FUNCTION "GESTIONE_ES" : VOID
TITLE =
{ S7_language := '9(1) Inglese (Stati Uniti)  21.12.2021  10:54:11' }
VERSION : 0.1


VAR_TEMP
  RETVAL : INT ;
END_VAR
BEGIN
NETWORK
TITLE =**************************************

NETWORK
TITLE =Abilita Gestione Risparmio Energetico
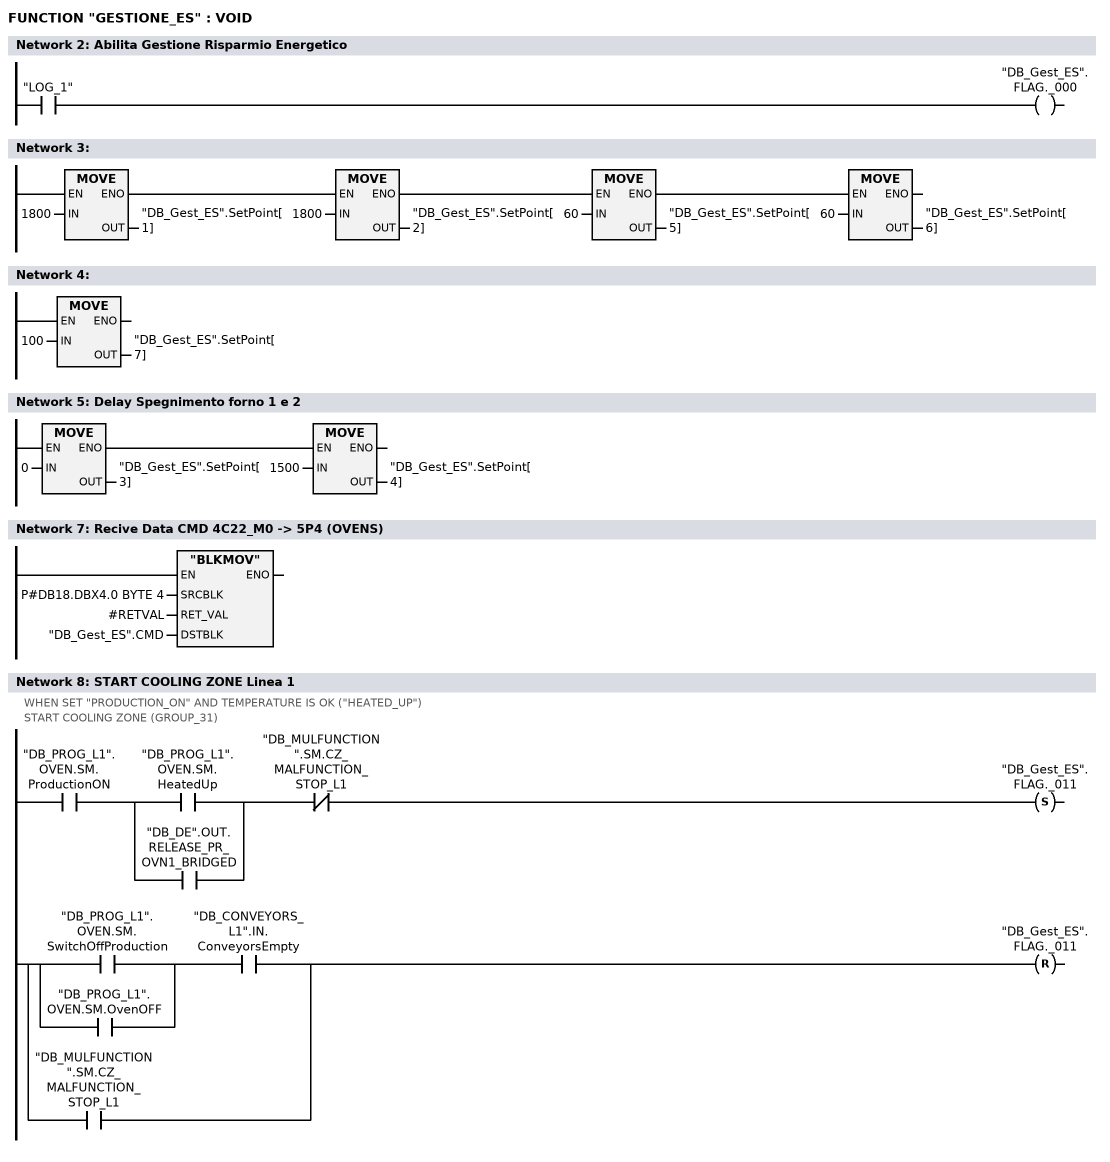
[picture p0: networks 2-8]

      U     "LOG_1";
      =     "DB_Gest_ES".FLAG._000;
NETWORK
TITLE =

      U(    ;
      U(    ;
      U(    ;
      L     1800;
      T     "DB_Gest_ES".SetPoint[1];
      SET   ;
      SAVE  ;
      CLR   ;
      U     BIE;
      )     ;
      SPBNB _001;
      L     1800;
      T     "DB_Gest_ES".SetPoint[2];
      SET   ;
      SAVE  ;
      CLR   ;
_001: U     BIE;
      )     ;
      SPBNB _002;
      L     60;
      T     "DB_Gest_ES".SetPoint[5];
      SET   ;
      SAVE  ;
      CLR   ;
_002: U     BIE;
      )     ;
      SPBNB _003;
      L     60;
      T     "DB_Gest_ES".SetPoint[6];
_003: NOP   0;
NETWORK
TITLE =

      L     100;
      T     "DB_Gest_ES".SetPoint[7];
      NOP   0;
NETWORK
TITLE =Delay Spegnimento forno 1 e 2

      U(    ;
      L     0;
      T     "DB_Gest_ES".SetPoint[3];
      SET   ;
      SAVE  ;
      CLR   ;
      U     BIE;
      )     ;
      SPBNB _004;
      L     1500;
      T     "DB_Gest_ES".SetPoint[4];
_004: NOP   0;
NETWORK
TITLE =**************************************

NETWORK
TITLE =Recive Data CMD 4C22_M0 -> 5P4 (OVENS)

      CALL "BLKMOV" (
           SRCBLK                   := P#DB18.DBX4.0 BYTE 4,
           RET_VAL                  := #RETVAL,
           DSTBLK                   := "DB_Gest_ES".CMD);
      NOP   0;
NETWORK
TITLE =START COOLING ZONE Linea 1
//WHEN SET "PRODUCTION_ON" AND TEMPERATURE IS OK ("HEATED_UP")
//START COOLING ZONE (GROUP_31)
      U     "DB_PROG_L1".OVEN.SM.ProductionON;
      U(    ;
      O     "DB_PROG_L1".OVEN.SM.HeatedUp;
      O     "DB_DE".OUT.RELEASE_PR_OVN1_BRIDGED;
      )     ;
      UN    "DB_MULFUNCTION".SM.CZ_MALFUNCTION_STOP_L1;
      S     "DB_Gest_ES".FLAG._011;
      U(    ;
      U(    ;
      O     "DB_PROG_L1".OVEN.SM.SwitchOffProduction;
      O     "DB_PROG_L1".OVEN.SM.OvenOFF;
      )     ;
      U     "DB_CONVEYORS_L1".IN.ConveyorsEmpty;
      O     "DB_MULFUNCTION".SM.CZ_MALFUNCTION_STOP_L1;
      )     ;
      R     "DB_Gest_ES".FLAG._011;
      NOP   0;
NETWORK
TITLE =Stop Raffreddamento Linea 1
//DB8.DBD38
      U     "DB_Gest_ES".FLAG._011;
      U     "DB_Gest_ES".FLAG._000;
      =     L      2.0;
      U     L      2.0;
      U(    ;
      U     "DB_Gest_ES".CMD.StopVentilazione_Zona1;
      UN    "DB_Gest_ES".FLAG._013;
      O     ;
      U     "DB_Gest_ES".Tmr.EN_Delay_01;
      UN    "DB_Gest_ES".Tmr.DN_Delay_01;
      )     ;
      S     "DB_Gest_ES".FLAG._001;
      U     L      2.0;
      UN    "DB_Gest_ES".CMD.StopVentilazione_Zona1;
      UN    "DB_Gest_ES".FLAG._013;
      S     "DB_Gest_ES".FLAG._013;
      U(    ;
      U     L      2.0;
      U     "DB_Gest_ES".CMD.VentilazioneRid_Zona1;
      =     "DB_Gest_ES".Tmr.EN_Delay_05;
      U     "DB_Gest_ES".Tmr.EN_Delay_05;
      )     ;
      U     "DB_Gest_ES".Tmr.DN_Delay_05;
      =     "DB_Gest_ES".FLAG._021;
NETWORK
TITLE =AUX Start Raff. Linea 1
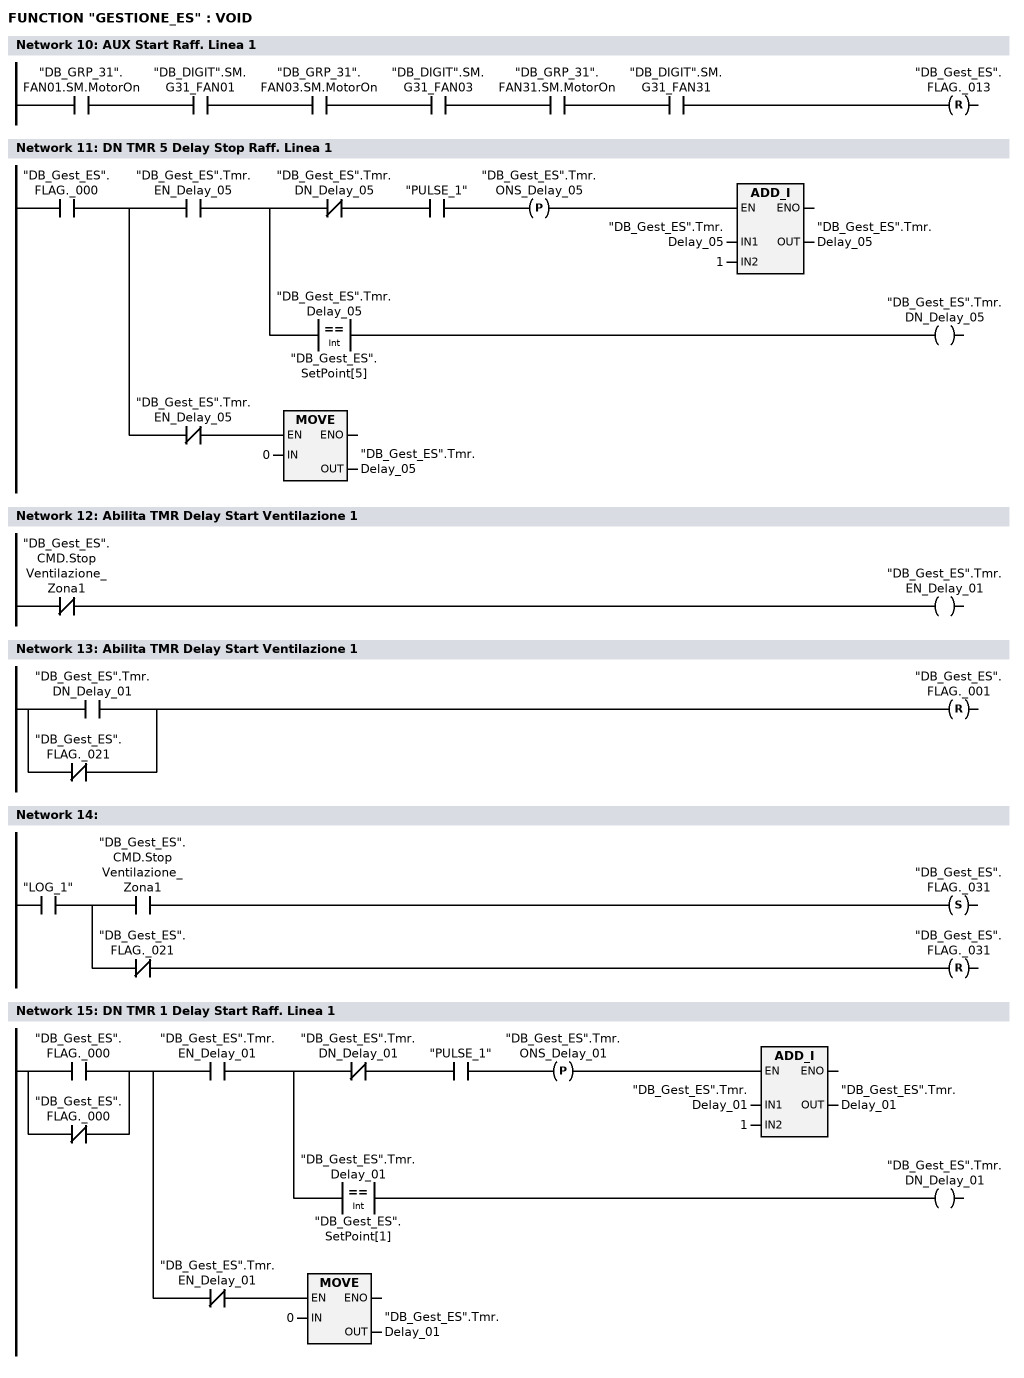
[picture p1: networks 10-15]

      U     "DB_GRP_31".FAN01.SM.MotorOn;
      U     "DB_DIGIT".SM.G31_FAN01;
      U     "DB_GRP_31".FAN03.SM.MotorOn;
      U     "DB_DIGIT".SM.G31_FAN03;
      U     "DB_GRP_31".FAN31.SM.MotorOn;
      U     "DB_DIGIT".SM.G31_FAN31;
      R     "DB_Gest_ES".FLAG._013;
NETWORK
TITLE =DN TMR 5 Delay Stop Raff. Linea 1

      U     "DB_Gest_ES".FLAG._000;
      =     L      2.0;
      U     L      2.0;
      U     "DB_Gest_ES".Tmr.EN_Delay_05;
      =     L      2.1;
      U     L      2.1;
      UN    "DB_Gest_ES".Tmr.DN_Delay_05;
      U     "PULSE_1";
      FP    "DB_Gest_ES".Tmr.ONS_Delay_05;
      SPBNB _005;
      L     "DB_Gest_ES".Tmr.Delay_05;
      L     1;
      +I    ;
      T     "DB_Gest_ES".Tmr.Delay_05;
_005: NOP   0;
      U     L      2.1;
      U(    ;
      L     "DB_Gest_ES".Tmr.Delay_05;
      L     "DB_Gest_ES".SetPoint[5];
      ==I   ;
      )     ;
      =     "DB_Gest_ES".Tmr.DN_Delay_05;
      U     L      2.0;
      UN    "DB_Gest_ES".Tmr.EN_Delay_05;
      SPBNB _006;
      L     0;
      T     "DB_Gest_ES".Tmr.Delay_05;
_006: NOP   0;
NETWORK
TITLE =Abilita TMR Delay Start Ventilazione 1

      UN    "DB_Gest_ES".CMD.StopVentilazione_Zona1;
      =     "DB_Gest_ES".Tmr.EN_Delay_01;
NETWORK
TITLE =Abilita TMR Delay Start Ventilazione 1

      O     "DB_Gest_ES".Tmr.DN_Delay_01;
      ON    "DB_Gest_ES".FLAG._021;
      R     "DB_Gest_ES".FLAG._001;
NETWORK
TITLE =

      U     "LOG_1";
      =     L      2.0;
      U     L      2.0;
      U     "DB_Gest_ES".CMD.StopVentilazione_Zona1;
      S     "DB_Gest_ES".FLAG._031;
      U     L      2.0;
      UN    "DB_Gest_ES".FLAG._021;
      R     "DB_Gest_ES".FLAG._031;
NETWORK
TITLE =DN TMR 1 Delay Start Raff. Linea 1

      O     "DB_Gest_ES".FLAG._000;
      ON    "DB_Gest_ES".FLAG._000;
      =     L      2.0;
      U     L      2.0;
      U     "DB_Gest_ES".Tmr.EN_Delay_01;
      =     L      2.1;
      U     L      2.1;
      UN    "DB_Gest_ES".Tmr.DN_Delay_01;
      U     "PULSE_1";
      FP    "DB_Gest_ES".Tmr.ONS_Delay_01;
      SPBNB _007;
      L     "DB_Gest_ES".Tmr.Delay_01;
      L     1;
      +I    ;
      T     "DB_Gest_ES".Tmr.Delay_01;
_007: NOP   0;
      U     L      2.1;
      U(    ;
      L     "DB_Gest_ES".Tmr.Delay_01;
      L     "DB_Gest_ES".SetPoint[1];
      ==I   ;
      )     ;
      =     "DB_Gest_ES".Tmr.DN_Delay_01;
      U     L      2.0;
      UN    "DB_Gest_ES".Tmr.EN_Delay_01;
      SPBNB _008;
      L     0;
      T     "DB_Gest_ES".Tmr.Delay_01;
_008: NOP   0;
NETWORK
TITLE =Stop Riscaldamento Linea 1

      U     "LOG_1";
      =     L      2.0;
      U(    ;
      U     L      2.0;
      U     "DB_Gest_ES".FLAG._000;
      U     "DB_CalendarioF1".CMD_OFF;
      U     "DB_CalendarioF1".Auto;
      UN    "DB_PROG_L1".OVEN.SM.SwitchOffProduction;
      U     "DB_Gest_ES".CMD.Stop_Riscarldo_Forno1;
      U     "DB_Gest_ES".CMD.AssenzaScoccheCabina;
      =     "DB_Gest_ES".Tmr.EN_Delay_03;
      U     "DB_Gest_ES".Tmr.EN_Delay_03;
      )     ;
      U     "DB_Gest_ES".Tmr.DN_Delay_03;
      S     "DB_Gest_ES".FLAG._003;
      R     "DB_CalendarioF1".CMD_OFF;
      U     L      2.0;
      U(    ;
      O     "DB_PROG_L1".OVEN.SM.SwitchOffProduction;
      O     "DB_PROG_L1".OVEN.SM.OvenOFF;
      O     "DB_PROG_L1".OVEN.CTRL.PreHeatingOn;
      O     "DB_PROG_L1".OVEN.CTRL.ProductionOn;
      )     ;
      R     "DB_Gest_ES".FLAG._003;
NETWORK
TITLE =DN TMR 3 Delay Stop Riscaldamento Linea 1
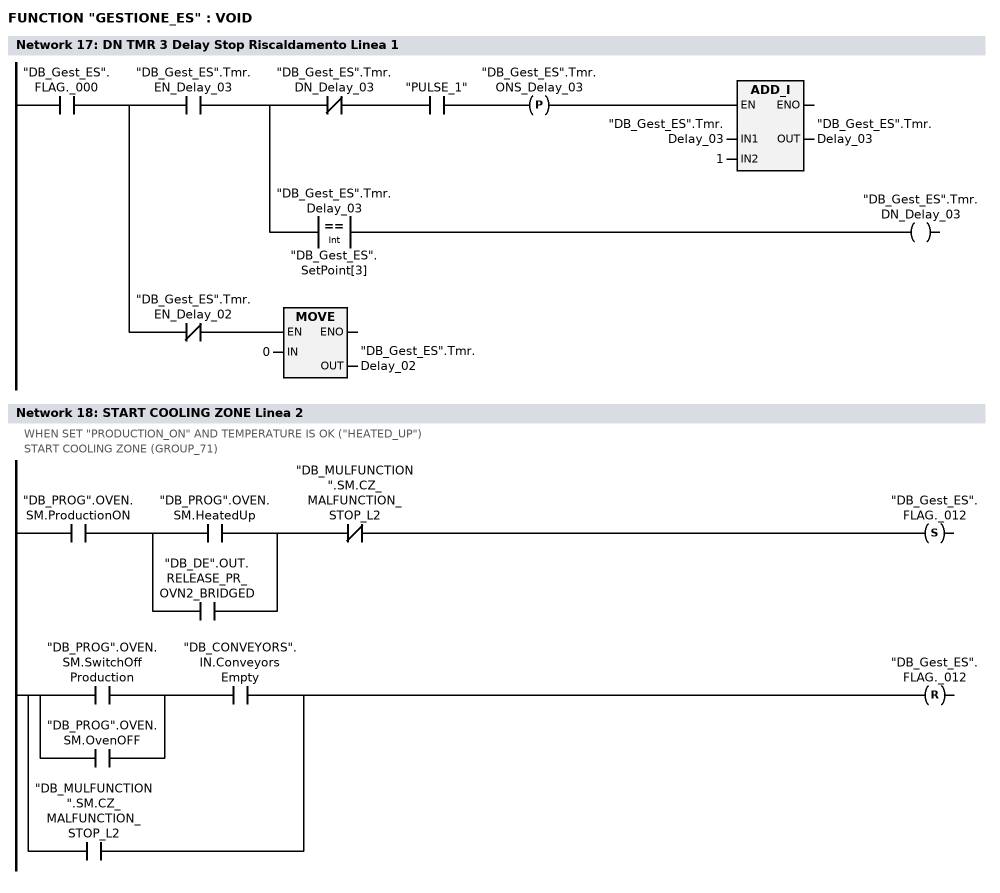
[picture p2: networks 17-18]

      U     "DB_Gest_ES".FLAG._000;
      =     L      2.0;
      U     L      2.0;
      U     "DB_Gest_ES".Tmr.EN_Delay_03;
      =     L      2.1;
      U     L      2.1;
      UN    "DB_Gest_ES".Tmr.DN_Delay_03;
      U     "PULSE_1";
      FP    "DB_Gest_ES".Tmr.ONS_Delay_03;
      SPBNB _009;
      L     "DB_Gest_ES".Tmr.Delay_03;
      L     1;
      +I    ;
      T     "DB_Gest_ES".Tmr.Delay_03;
_009: NOP   0;
      U     L      2.1;
      U(    ;
      L     "DB_Gest_ES".Tmr.Delay_03;
      L     "DB_Gest_ES".SetPoint[3];
      ==I   ;
      )     ;
      =     "DB_Gest_ES".Tmr.DN_Delay_03;
      U     L      2.0;
      UN    "DB_Gest_ES".Tmr.EN_Delay_02;
      SPBNB _00a;
      L     0;
      T     "DB_Gest_ES".Tmr.Delay_02;
_00a: NOP   0;
NETWORK
TITLE =START COOLING ZONE Linea 2
//WHEN SET "PRODUCTION_ON" AND TEMPERATURE IS OK ("HEATED_UP")
//START COOLING ZONE (GROUP_71)
      U     "DB_PROG".OVEN.SM.ProductionON;
      U(    ;
      O     "DB_PROG".OVEN.SM.HeatedUp;
      O     "DB_DE".OUT.RELEASE_PR_OVN2_BRIDGED;
      )     ;
      UN    "DB_MULFUNCTION".SM.CZ_MALFUNCTION_STOP_L2;
      S     "DB_Gest_ES".FLAG._012;
      U(    ;
      U(    ;
      O     "DB_PROG".OVEN.SM.SwitchOffProduction;
      O     "DB_PROG".OVEN.SM.OvenOFF;
      )     ;
      U     "DB_CONVEYORS".IN.ConveyorsEmpty;
      O     "DB_MULFUNCTION".SM.CZ_MALFUNCTION_STOP_L2;
      )     ;
      R     "DB_Gest_ES".FLAG._012;
      NOP   0;
NETWORK
TITLE =Stop Raffreddamento Linea 2
//DB8.DBD38
      U     "DB_Gest_ES".FLAG._012;
      U     "DB_Gest_ES".FLAG._000;
      =     L      2.0;
      U     L      2.0;
      U(    ;
      U     "DB_Gest_ES".CMD.StopVentilazione_Zona2;
      UN    "DB_Gest_ES".FLAG._014;
      O     ;
      U     "DB_Gest_ES".Tmr.EN_Delay_02;
      UN    "DB_Gest_ES".Tmr.DN_Delay_02;
      )     ;
      S     "DB_Gest_ES".FLAG._002;
      U     L      2.0;
      UN    "DB_Gest_ES".CMD.StopVentilazione_Zona2;
      UN    "DB_Gest_ES".FLAG._014;
      S     "DB_Gest_ES".FLAG._014;
      U(    ;
      U     L      2.0;
      U     "DB_Gest_ES".CMD.VentilazioneRid_Zona2;
      =     "DB_Gest_ES".Tmr.EN_Delay_06;
      U     "DB_Gest_ES".Tmr.EN_Delay_06;
      )     ;
      U     "DB_Gest_ES".Tmr.DN_Delay_06;
      =     "DB_Gest_ES".FLAG._022;
NETWORK
TITLE =AUX Start Raff. Linea 2
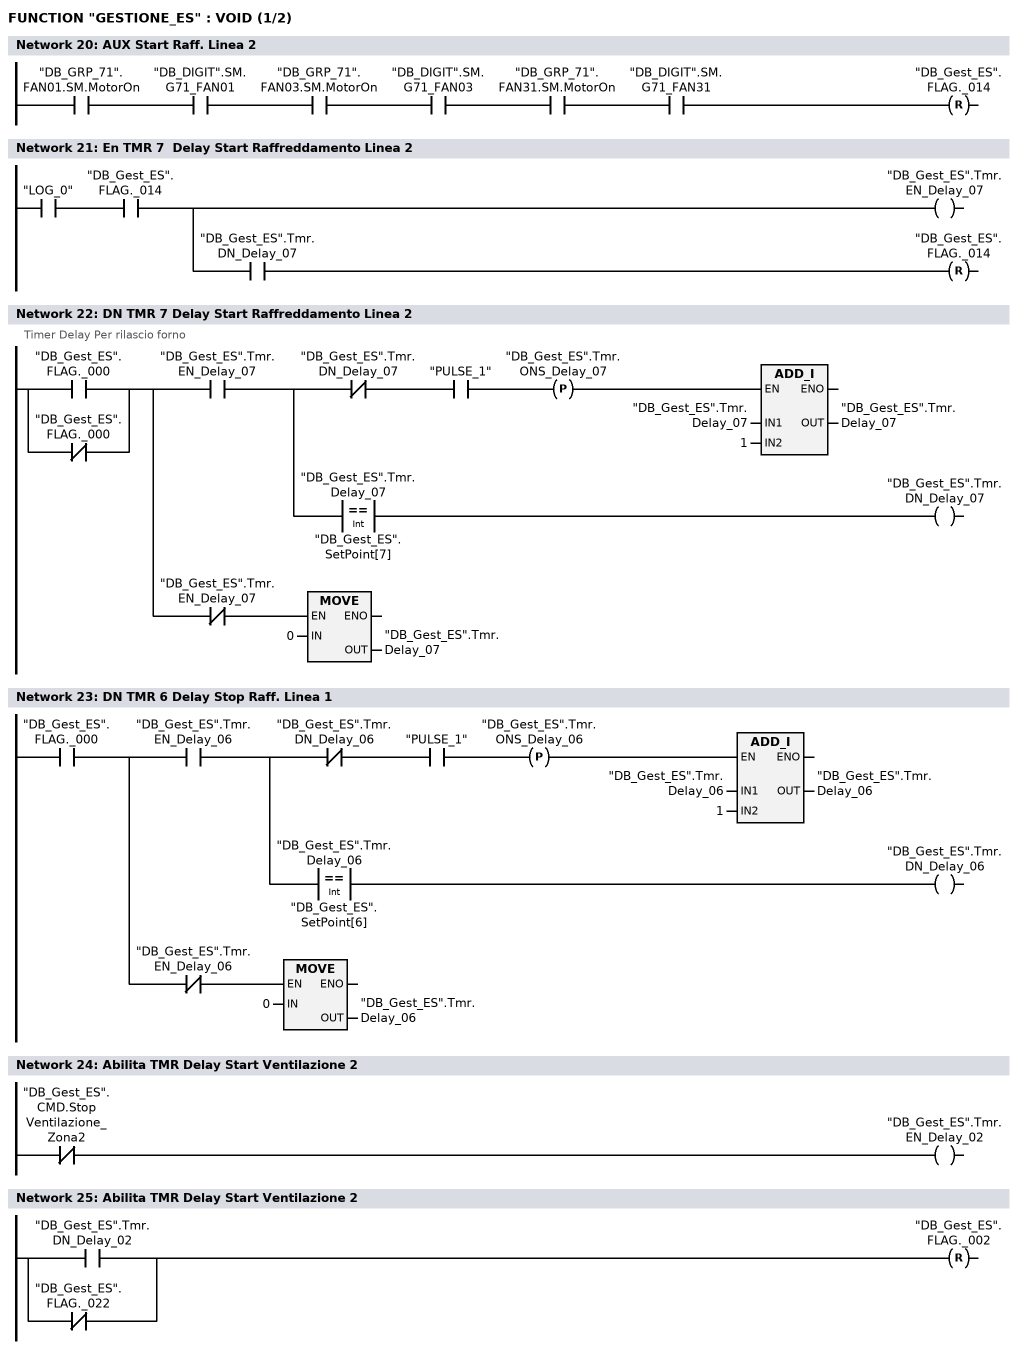
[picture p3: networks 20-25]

      U     "DB_GRP_71".FAN01.SM.MotorOn;
      U     "DB_DIGIT".SM.G71_FAN01;
      U     "DB_GRP_71".FAN03.SM.MotorOn;
      U     "DB_DIGIT".SM.G71_FAN03;
      U     "DB_GRP_71".FAN31.SM.MotorOn;
      U     "DB_DIGIT".SM.G71_FAN31;
      R     "DB_Gest_ES".FLAG._014;
NETWORK
TITLE =En TMR 7  Delay Start Raffreddamento Linea 2

      U     "LOG_0";
      U     "DB_Gest_ES".FLAG._014;
      =     L      2.0;
      U     L      2.0;
      BLD   102;
      =     "DB_Gest_ES".Tmr.EN_Delay_07;
      U     L      2.0;
      U     "DB_Gest_ES".Tmr.DN_Delay_07;
      R     "DB_Gest_ES".FLAG._014;
NETWORK
TITLE =DN TMR 7 Delay Start Raffreddamento Linea 2
//Timer Delay Per rilascio forno
      O     "DB_Gest_ES".FLAG._000;
      ON    "DB_Gest_ES".FLAG._000;
      =     L      2.0;
      U     L      2.0;
      U     "DB_Gest_ES".Tmr.EN_Delay_07;
      =     L      2.1;
      U     L      2.1;
      UN    "DB_Gest_ES".Tmr.DN_Delay_07;
      U     "PULSE_1";
      FP    "DB_Gest_ES".Tmr.ONS_Delay_07;
      SPBNB _00b;
      L     "DB_Gest_ES".Tmr.Delay_07;
      L     1;
      +I    ;
      T     "DB_Gest_ES".Tmr.Delay_07;
_00b: NOP   0;
      U     L      2.1;
      U(    ;
      L     "DB_Gest_ES".Tmr.Delay_07;
      L     "DB_Gest_ES".SetPoint[7];
      ==I   ;
      )     ;
      =     "DB_Gest_ES".Tmr.DN_Delay_07;
      U     L      2.0;
      UN    "DB_Gest_ES".Tmr.EN_Delay_07;
      SPBNB _00c;
      L     0;
      T     "DB_Gest_ES".Tmr.Delay_07;
_00c: NOP   0;
NETWORK
TITLE =DN TMR 6 Delay Stop Raff. Linea 1

      U     "DB_Gest_ES".FLAG._000;
      =     L      2.0;
      U     L      2.0;
      U     "DB_Gest_ES".Tmr.EN_Delay_06;
      =     L      2.1;
      U     L      2.1;
      UN    "DB_Gest_ES".Tmr.DN_Delay_06;
      U     "PULSE_1";
      FP    "DB_Gest_ES".Tmr.ONS_Delay_06;
      SPBNB _00d;
      L     "DB_Gest_ES".Tmr.Delay_06;
      L     1;
      +I    ;
      T     "DB_Gest_ES".Tmr.Delay_06;
_00d: NOP   0;
      U     L      2.1;
      U(    ;
      L     "DB_Gest_ES".Tmr.Delay_06;
      L     "DB_Gest_ES".SetPoint[6];
      ==I   ;
      )     ;
      =     "DB_Gest_ES".Tmr.DN_Delay_06;
      U     L      2.0;
      UN    "DB_Gest_ES".Tmr.EN_Delay_06;
      SPBNB _00e;
      L     0;
      T     "DB_Gest_ES".Tmr.Delay_06;
_00e: NOP   0;
NETWORK
TITLE =Abilita TMR Delay Start Ventilazione 2

      UN    "DB_Gest_ES".CMD.StopVentilazione_Zona2;
      =     "DB_Gest_ES".Tmr.EN_Delay_02;
NETWORK
TITLE =Abilita TMR Delay Start Ventilazione 2

      O     "DB_Gest_ES".Tmr.DN_Delay_02;
      ON    "DB_Gest_ES".FLAG._022;
      R     "DB_Gest_ES".FLAG._002;
NETWORK
TITLE =DN TMR 2 Delay Stop Riscaldamento Linea 2
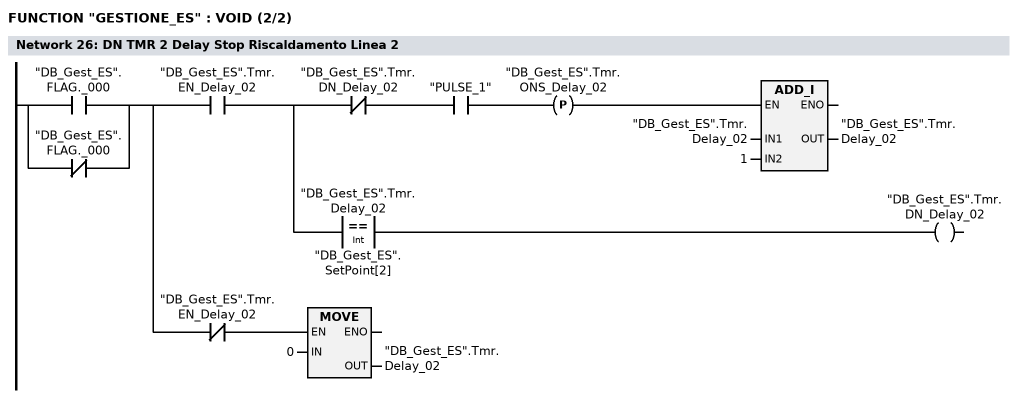
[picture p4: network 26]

      O     "DB_Gest_ES".FLAG._000;
      ON    "DB_Gest_ES".FLAG._000;
      =     L      2.0;
      U     L      2.0;
      U     "DB_Gest_ES".Tmr.EN_Delay_02;
      =     L      2.1;
      U     L      2.1;
      UN    "DB_Gest_ES".Tmr.DN_Delay_02;
      U     "PULSE_1";
      FP    "DB_Gest_ES".Tmr.ONS_Delay_02;
      SPBNB _00f;
      L     "DB_Gest_ES".Tmr.Delay_02;
      L     1;
      +I    ;
      T     "DB_Gest_ES".Tmr.Delay_02;
_00f: NOP   0;
      U     L      2.1;
      U(    ;
      L     "DB_Gest_ES".Tmr.Delay_02;
      L     "DB_Gest_ES".SetPoint[2];
      ==I   ;
      )     ;
      =     "DB_Gest_ES".Tmr.DN_Delay_02;
      U     L      2.0;
      UN    "DB_Gest_ES".Tmr.EN_Delay_02;
      SPBNB _010;
      L     0;
      T     "DB_Gest_ES".Tmr.Delay_02;
_010: NOP   0;
NETWORK
TITLE =Stop Riscaldamento Linea 2

      U     "LOG_1";
      =     L      2.0;
      U(    ;
      U     L      2.0;
      U     "DB_Gest_ES".FLAG._000;
      U     "DB_CalendarioF2".CMD_OFF;
      U     "DB_CalendarioF2".Auto;
      UN    "DB_PROG".OVEN.SM.SwitchOffProduction;
      U     "DB_Gest_ES".CMD.AssenzaScoccheCabina;
      =     "DB_Gest_ES".Tmr.EN_Delay_04;
      U     "DB_Gest_ES".Tmr.EN_Delay_04;
      )     ;
      U     "DB_Gest_ES".CMD.Stop_Riscarldo_Forno2;
      U     "DB_Gest_ES".Tmr.DN_Delay_04;
      S     "DB_Gest_ES".FLAG._004;
      R     "DB_CalendarioF2".CMD_OFF;
      U     L      2.0;
      U(    ;
      O     "DB_PROG".OVEN.SM.SwitchOffProduction;
      O     "DB_PROG".OVEN.SM.OvenOFF;
      O     "DB_PROG".OVEN.CTRL.PreHeatingOn;
      O     "DB_PROG".OVEN.CTRL.ProductionOn;
      )     ;
      R     "DB_Gest_ES".FLAG._004;
NETWORK
TITLE =DN TMR 4 Delay Stop Riscaldamento Linea 1
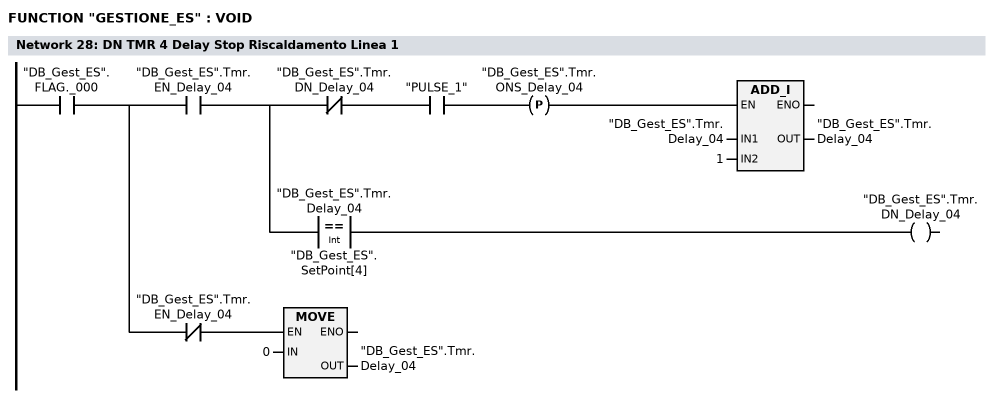
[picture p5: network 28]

      U     "DB_Gest_ES".FLAG._000;
      =     L      2.0;
      U     L      2.0;
      U     "DB_Gest_ES".Tmr.EN_Delay_04;
      =     L      2.1;
      U     L      2.1;
      UN    "DB_Gest_ES".Tmr.DN_Delay_04;
      U     "PULSE_1";
      FP    "DB_Gest_ES".Tmr.ONS_Delay_04;
      SPBNB _011;
      L     "DB_Gest_ES".Tmr.Delay_04;
      L     1;
      +I    ;
      T     "DB_Gest_ES".Tmr.Delay_04;
_011: NOP   0;
      U     L      2.1;
      U(    ;
      L     "DB_Gest_ES".Tmr.Delay_04;
      L     "DB_Gest_ES".SetPoint[4];
      ==I   ;
      )     ;
      =     "DB_Gest_ES".Tmr.DN_Delay_04;
      U     L      2.0;
      UN    "DB_Gest_ES".Tmr.EN_Delay_04;
      SPBNB _012;
      L     0;
      T     "DB_Gest_ES".Tmr.Delay_04;
_012: NOP   0;
NETWORK
TITLE =**************************************

NETWORK
TITLE =######################################

NETWORK
TITLE =Send Data CMD 5P4 -> 4C22_M0

NETWORK
TITLE =######################################

NETWORK
TITLE =#CALENDARIO FORNO 1

NETWORK
TITLE =Set

//Anno
      L     DB3100.DBB    8;
      T     "DB_CalendarioF1".PLC.Year;
//Mese
      L     DB3100.DBB    9;
      T     "DB_CalendarioF1".PLC.Mon;
//Giorno
      L     DB3100.DBB   10;
      T     "DB_CalendarioF1".PLC.Day;


//Ore
      L     DB3100.DBB   11;
      BTI   ;
      T     "DB_CalendarioF1".PLC.Hour;
//Minuti
      L     DB3100.DBB   12;
      BTI   ;
      T     "DB_CalendarioF1".PLC.Min;



NETWORK
TITLE =Calcolo del giorno della settimana

      L     DB3100.DBB   15;
      UW    W#16#F;
      T     "DB_CalendarioF1".PLC.WeekDay;
NETWORK
TITLE =Richiamo FC Gestione calendario
//P#DB101.DBX 50.0 BYTE 4
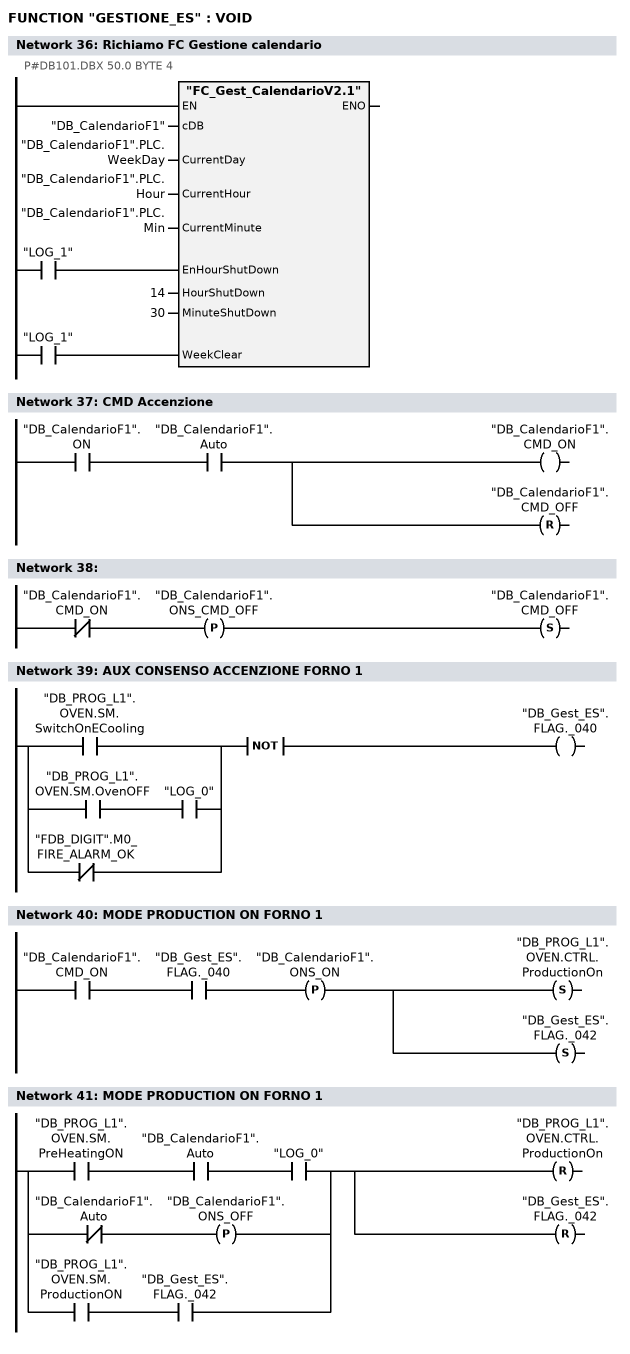
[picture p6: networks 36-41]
      U     "LOG_1";
      =     L      2.0;
      BLD   103;
      U     "LOG_1";
      =     L      2.1;
      BLD   103;
      CALL "FC_Gest_CalendarioV2.1" (
           cDB                      := "DB_CalendarioF1",
           CurrentDay               := "DB_CalendarioF1".PLC.WeekDay,
           CurrentHour              := "DB_CalendarioF1".PLC.Hour,
           CurrentMinute            := "DB_CalendarioF1".PLC.Min,
           EnHourShutDown           := L      2.0,
           HourShutDown             := 14,
           MinuteShutDown           := 30,
           WeekClear                := L      2.1);
      NOP   0;
NETWORK
TITLE =CMD Accenzione

      U     "DB_CalendarioF1".ON;
      U     "DB_CalendarioF1".Auto;
      =     "DB_CalendarioF1".CMD_ON;
      R     "DB_CalendarioF1".CMD_OFF;
NETWORK
TITLE =

      UN    "DB_CalendarioF1".CMD_ON;
      FP    "DB_CalendarioF1".ONS_CMD_OFF;
      S     "DB_CalendarioF1".CMD_OFF;
NETWORK
TITLE =AUX CONSENSO ACCENZIONE FORNO 1

      U(    ;
      O     "DB_PROG_L1".OVEN.SM.SwitchOnECooling;
      O     ;
      U     "DB_PROG_L1".OVEN.SM.OvenOFF;
      U     "LOG_0";
      ON    "FDB_DIGIT".M0_FIRE_ALARM_OK;
      )     ;
      NOT   ;
      =     "DB_Gest_ES".FLAG._040;
NETWORK
TITLE =MODE PRODUCTION ON FORNO 1

      U     "DB_CalendarioF1".CMD_ON;
      U     "DB_Gest_ES".FLAG._040;
      FP    "DB_CalendarioF1".ONS_ON;
      S     "DB_PROG_L1".OVEN.CTRL.ProductionOn;
      S     "DB_Gest_ES".FLAG._042;
NETWORK
TITLE =MODE PRODUCTION ON FORNO 1

      U     "DB_PROG_L1".OVEN.SM.PreHeatingON;
      U     "DB_CalendarioF1".Auto;
      U     "LOG_0";
      O(    ;
      UN    "DB_CalendarioF1".Auto;
      FP    "DB_CalendarioF1".ONS_OFF;
      )     ;
      O     ;
      U     "DB_PROG_L1".OVEN.SM.ProductionON;
      U     "DB_Gest_ES".FLAG._042;
      R     "DB_PROG_L1".OVEN.CTRL.ProductionOn;
      R     "DB_Gest_ES".FLAG._042;
NETWORK
TITLE =######################################

NETWORK
TITLE =#CALENDARIO FORNO 2

NETWORK
TITLE =Set

//Anno
      L     DB3100.DBB    8;
      T     "DB_CalendarioF2".PLC.Year;
//Mese
      L     DB3100.DBB    9;
      T     "DB_CalendarioF2".PLC.Mon;
//Giorno
      L     DB3100.DBB   10;
      T     "DB_CalendarioF2".PLC.Day;


//Ore
      L     DB3100.DBB   11;
      BTI   ;
      T     "DB_CalendarioF2".PLC.Hour;
//Minuti
      L     DB3100.DBB   12;
      BTI   ;
      T     "DB_CalendarioF2".PLC.Min;



NETWORK
TITLE =Calcolo del giorno della settimana

      L     DB3100.DBB   15;
      UW    W#16#F;
      T     "DB_CalendarioF2".PLC.WeekDay;
NETWORK
TITLE =Richiamo FC Gestione calendario
//P#DB101.DBX 50.0 BYTE 4
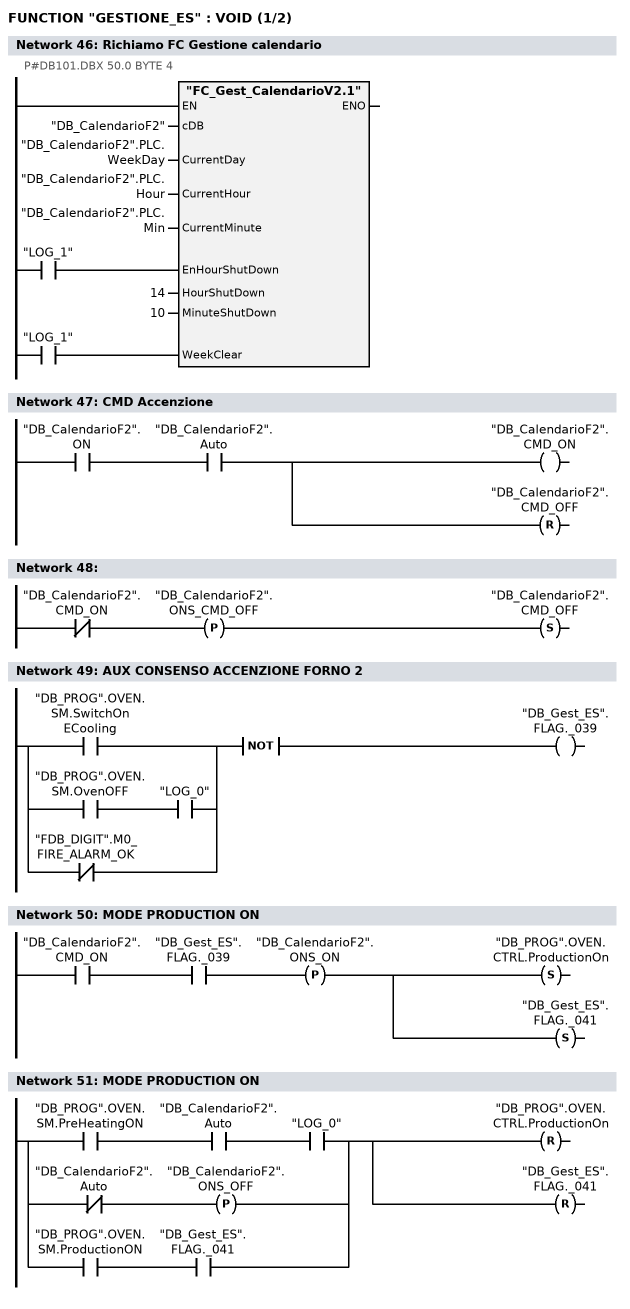
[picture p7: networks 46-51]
      U     "LOG_1";
      =     L      2.0;
      BLD   103;
      U     "LOG_1";
      =     L      2.1;
      BLD   103;
      CALL "FC_Gest_CalendarioV2.1" (
           cDB                      := "DB_CalendarioF2",
           CurrentDay               := "DB_CalendarioF2".PLC.WeekDay,
           CurrentHour              := "DB_CalendarioF2".PLC.Hour,
           CurrentMinute            := "DB_CalendarioF2".PLC.Min,
           EnHourShutDown           := L      2.0,
           HourShutDown             := 14,
           MinuteShutDown           := 10,
           WeekClear                := L      2.1);
      NOP   0;
NETWORK
TITLE =CMD Accenzione

      U     "DB_CalendarioF2".ON;
      U     "DB_CalendarioF2".Auto;
      =     "DB_CalendarioF2".CMD_ON;
      R     "DB_CalendarioF2".CMD_OFF;
NETWORK
TITLE =

      UN    "DB_CalendarioF2".CMD_ON;
      FP    "DB_CalendarioF2".ONS_CMD_OFF;
      S     "DB_CalendarioF2".CMD_OFF;
NETWORK
TITLE =AUX CONSENSO ACCENZIONE FORNO 2

      U(    ;
      O     "DB_PROG".OVEN.SM.SwitchOnECooling;
      O     ;
      U     "DB_PROG".OVEN.SM.OvenOFF;
      U     "LOG_0";
      ON    "FDB_DIGIT".M0_FIRE_ALARM_OK;
      )     ;
      NOT   ;
      =     "DB_Gest_ES".FLAG._039;
NETWORK
TITLE =MODE PRODUCTION ON

      U     "DB_CalendarioF2".CMD_ON;
      U     "DB_Gest_ES".FLAG._039;
      FP    "DB_CalendarioF2".ONS_ON;
      S     "DB_PROG".OVEN.CTRL.ProductionOn;
      S     "DB_Gest_ES".FLAG._041;
NETWORK
TITLE =MODE PRODUCTION ON

      U     "DB_PROG".OVEN.SM.PreHeatingON;
      U     "DB_CalendarioF2".Auto;
      U     "LOG_0";
      O(    ;
      UN    "DB_CalendarioF2".Auto;
      FP    "DB_CalendarioF2".ONS_OFF;
      )     ;
      O     ;
      U     "DB_PROG".OVEN.SM.ProductionON;
      U     "DB_Gest_ES".FLAG._041;
      R     "DB_PROG".OVEN.CTRL.ProductionOn;
      R     "DB_Gest_ES".FLAG._041;
NETWORK
TITLE =######################################

NETWORK
TITLE =CABINA PRIMER

NETWORK
TITLE =AUX CONSENSO ACCENZIONE PRIMER
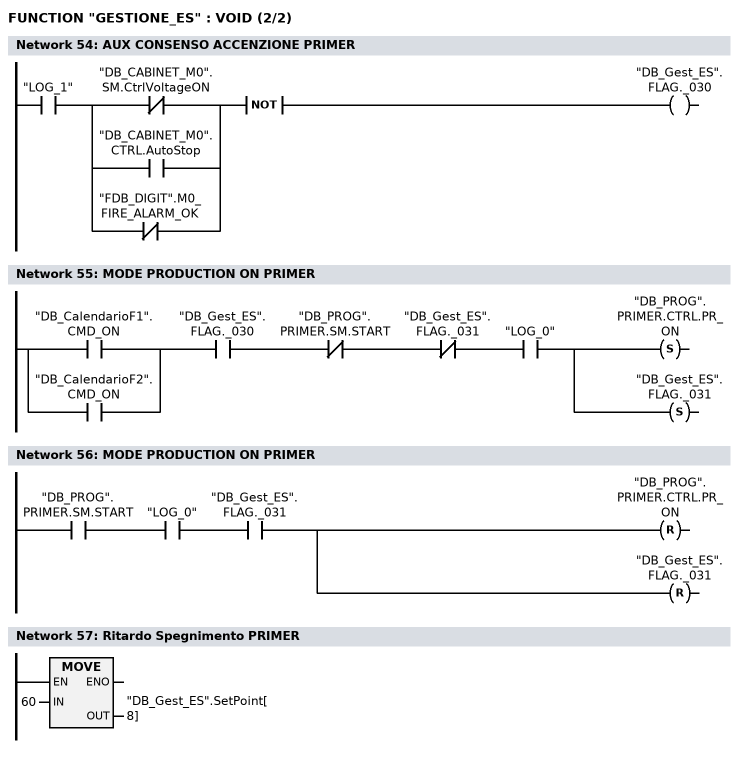
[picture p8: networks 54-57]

      U     "LOG_1";
      U(    ;
      ON    "DB_CABINET_M0".SM.CtrlVoltageON;
      O     "DB_CABINET_M0".CTRL.AutoStop;
      ON    "FDB_DIGIT".M0_FIRE_ALARM_OK;
      )     ;
      NOT   ;
      =     "DB_Gest_ES".FLAG._030;
NETWORK
TITLE =MODE PRODUCTION ON PRIMER

      U(    ;
      O     "DB_CalendarioF1".CMD_ON;
      O     "DB_CalendarioF2".CMD_ON;
      )     ;
      U     "DB_Gest_ES".FLAG._030;
      UN    "DB_PROG".PRIMER.SM.START;
      UN    "DB_Gest_ES".FLAG._031;
      U     "LOG_0";
      S     "DB_PROG".PRIMER.CTRL.PR_ON;
      S     "DB_Gest_ES".FLAG._031;
NETWORK
TITLE =MODE PRODUCTION ON PRIMER

      U     "DB_PROG".PRIMER.SM.START;
      U     "LOG_0";
      U     "DB_Gest_ES".FLAG._031;
      R     "DB_PROG".PRIMER.CTRL.PR_ON;
      R     "DB_Gest_ES".FLAG._031;
NETWORK
TITLE =Ritardo Spegnimento PRIMER

      L     60;
      T     "DB_Gest_ES".SetPoint[8];
      NOP   0;
NETWORK
TITLE =Stop CABINA PRIMER

      U     "LOG_1";
      =     L      2.0;
      U(    ;
      U     L      2.0;
      U     "DB_Gest_ES".FLAG._000;
      U     "DB_PROG".PRIMER.SM.ON;
      UN    "DB_Gest_ES".FLAG._033;
      U     "DB_CalendarioF2".Auto;
      U     "DB_CalendarioF1".Auto;
      UN    "DB_CalendarioF1".CMD_ON;
      UN    "DB_CalendarioF2".CMD_ON;
      UN    "DB_PROG".OVEN.CTRL.ProductionOn;
      UN    "DB_PROG_L1".OVEN.CTRL.ProductionOn;
      U     "DB_Gest_ES".CMD.AssenzaScoccheCabina;
      =     "DB_Gest_ES".Tmr.EN_Delay_08;
      U     "DB_Gest_ES".Tmr.EN_Delay_08;
      )     ;
      U     "DB_Gest_ES".Tmr.DN_Delay_08;
      S     "DB_Gest_ES".FLAG._032;
      R     "DB_PROG".PRIMER.SM.ON;
      U     L      2.0;
      UN    "DB_PROG".PRIMER.SM.ON;
      U     "DB_Gest_ES".FLAG._032;
      R     "DB_Gest_ES".FLAG._032;
NETWORK
TITLE =DN TMR 4 Delay Stop Riscaldamento Linea 1
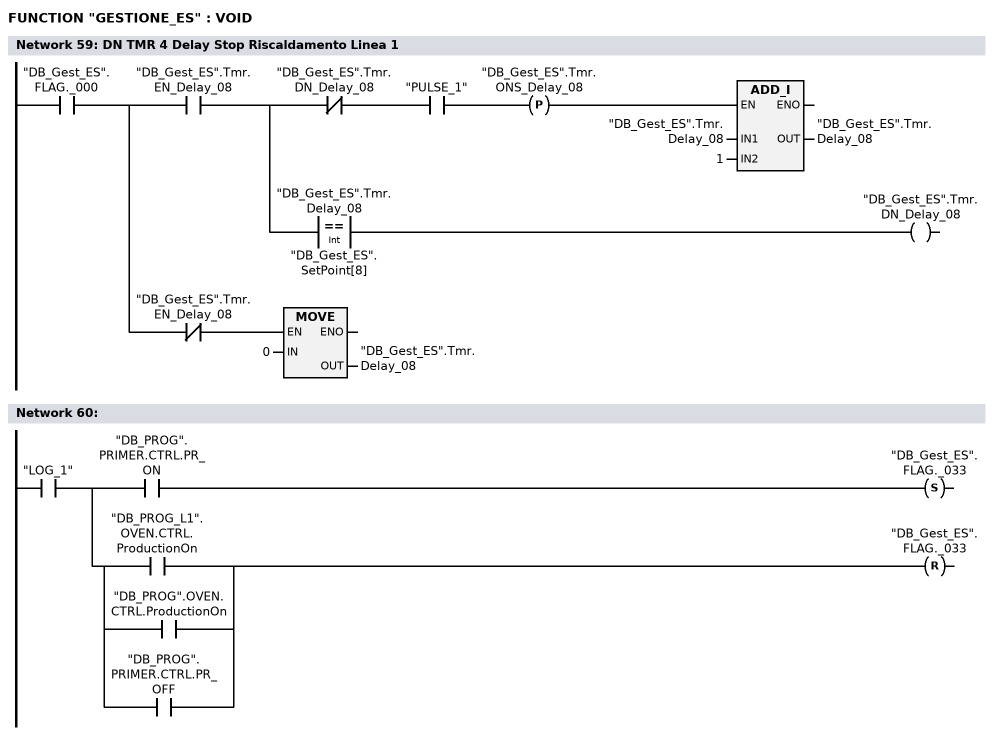
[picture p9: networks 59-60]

      U     "DB_Gest_ES".FLAG._000;
      =     L      2.0;
      U     L      2.0;
      U     "DB_Gest_ES".Tmr.EN_Delay_08;
      =     L      2.1;
      U     L      2.1;
      UN    "DB_Gest_ES".Tmr.DN_Delay_08;
      U     "PULSE_1";
      FP    "DB_Gest_ES".Tmr.ONS_Delay_08;
      SPBNB _013;
      L     "DB_Gest_ES".Tmr.Delay_08;
      L     1;
      +I    ;
      T     "DB_Gest_ES".Tmr.Delay_08;
_013: NOP   0;
      U     L      2.1;
      U(    ;
      L     "DB_Gest_ES".Tmr.Delay_08;
      L     "DB_Gest_ES".SetPoint[8];
      ==I   ;
      )     ;
      =     "DB_Gest_ES".Tmr.DN_Delay_08;
      U     L      2.0;
      UN    "DB_Gest_ES".Tmr.EN_Delay_08;
      SPBNB _014;
      L     0;
      T     "DB_Gest_ES".Tmr.Delay_08;
_014: NOP   0;
NETWORK
TITLE =

      U     "LOG_1";
      =     L      2.0;
      U     L      2.0;
      U     "DB_PROG".PRIMER.CTRL.PR_ON;
      S     "DB_Gest_ES".FLAG._033;
      U     L      2.0;
      U(    ;
      O     "DB_PROG_L1".OVEN.CTRL.ProductionOn;
      O     "DB_PROG".OVEN.CTRL.ProductionOn;
      O     "DB_PROG".PRIMER.CTRL.PR_OFF;
      )     ;
      R     "DB_Gest_ES".FLAG._033;
END_FUNCTION

